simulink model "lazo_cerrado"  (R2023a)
settings: Solver=VariableStepAuto  StartTime=0.0  StopTime=10.0  RelTol=1e-3
libraries: visiontextngfix x6, slpidlib x3

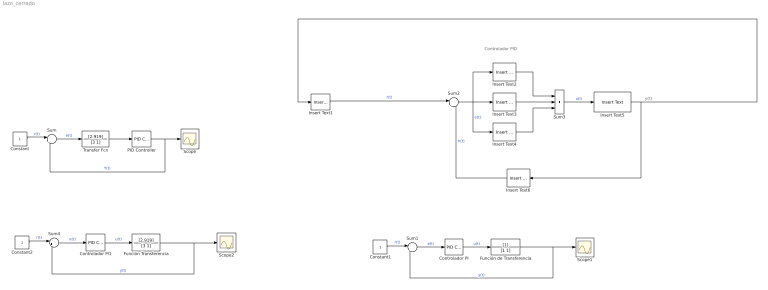
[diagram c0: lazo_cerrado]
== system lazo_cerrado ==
  note: Controlador PID
  note: y(t)
  Constant : Constant
  Constant1 : Constant
  Constant2 : Constant
  Controlador PI : slpidlib/PID Controller  Controller=PI  Form=Parallel  TimeDomain=Continuous-time  UseExternalTs=off  SampleTime=-1  IntegratorMethod=Forward Euler  FilterMethod=Forward Euler  ControllerParametersSource=internal  P=1  I=1  UseKiTs=off  D=0  N=100  UseFilter=on  TunerSelectOption=Transfer Function Based (PID Tuner App)  InitialConditionSource=internal  InitialConditionForIntegrator=0  InitialConditionForFilter=0  DifferentiatorICPrevScaledInput=0  ExternalReset=none  TrackingMode=off  Kt=1  LimitOutput=off  SatLimitsSource=internal  UpperSaturationLimit=inf  LowerSaturationLimit=-inf  LinearizeAsGain=on  AntiWindupMode=none  Kb=1  LimitIntegrator=off  UpperIntegratorSaturationLimit=inf  LowerIntegratorSaturationLimit=-inf  POutMin=[]  POutMax=[]  IOutMin=[]  IOutMax=[]  DOutMin=[]  DOutMax=[]  NOutMin=[]  NOutMax=[]  SumOutMin=[]  SumOutMax=[]  SaturationOutMin=[]  SaturationOutMax=[]  PParamMin=[]  PParamMax=[]  IParamMin=[]  IParamMax=[]  DParamMin=[]  DParamMax=[]  NParamMin=[]  NParamMax=[]  KbParamMin=[]  KbParamMax=[]  KtParamMin=[]  KtParamMax=[]  KbOutMin=[]  KbOutMax=[]  KtOutMin=[]  KtOutMax=[]  IntegratorOutMin=[]  IntegratorOutMax=[]  FilterOutMin=[]  FilterOutMax=[]  SumI1OutMin=[]  SumI1OutMax=[]  SumI2OutMin=[]  SumI2OutMax=[]  SumI3OutMin=[]  SumI3OutMax=[]  SumI4OutMin=[]  SumI4OutMax=[]  SumDOutMin=[]  SumDOutMax=[]  DifferentiatorOutMin=[]  DifferentiatorOutMax=[]  FilterDiffOutCoefMin=[]  FilterDiffOutCoefMax=[]  ReciprocalOutMin=[]  ReciprocalOutMax=[]  SumDenOutMin=[]  SumDenOutMax=[]  SumNumOutMin=[]  SumNumOutMax=[]  DivideOutMin=[]  DivideOutMax=[]  UdiffTsProdOutMin=[]  UdiffTsProdOutMax=[]  NTsProdOutMin=[]  NTsProdOutMax=[]  UintegralTsProdOutMin=[]  UintegralTsProdOutMax=[]  UngainTsProdOutMin=[]  UngainTsProdOutMax=[]  ClampingZeroOutDataTypeStr=Inherit: Inherit via back propagation  ClampingZeroOutMin=[]  ClampingZeroOutMax=[]  FilterDenConstantOutDataTypeStr=Inherit: Inherit via back propagation  FilterDenConstantOutMin=[]  FilterDenConstantOutMax=[]  PCopyOutDataTypeStr=Inherit: Inherit via back propagation  PCopyOutMin=[]  PCopyOutMax=[]  NCopyOutDataTypeStr=Inherit: Inherit via back propagation  NCopyOutMin=[]  NCopyOutMax=[]  IntegratorContinuousStateAttributes=''  IntegratorStateMustResolveToSignalObject=off  IntegratorRTWStateStorageClass=Auto  FilterContinuousStateAttributes=''  FilterStateMustResolveToSignalObject=off  FilterRTWStateStorageClass=Auto  ParallelPVariant=InternalParameters  IdealPVariant=Disabled  IVariant=InternalParameters  DVariant=Disabled  IntegratorVariant=Continuous  SatVariant=Disabled  AWVariant=Passthrough  PCopyVariant=Disabled  TRVariant=Disabled  FdbkBlocksVariant=Forward  IdealPFdbkVariant=Disabled  SatFdbkVariant=Disabled  DerivativeFilterVariant=Disabled  NVariant=Disabled  NCopyVariant=Disabled_SignalSpec  FilterICVariant=Disabled  IntegratorICVariant=InternalICs  ExternalResetVariant=Disabled  TRSumVariant=Passthrough  SumFdbkVariant=Disabled  SumVariant=Sum_PI  TsampFilterVariant=InternalTs  TsampNgainVariant=Passthrough  TsampIntegralVariant=Disabled_SignalSpec  ExternalSaturationOutDataTypeStr=Inherit: Same as second input
  Controlador PI1 : slpidlib/PID Controller  Controller=PI  Form=Parallel  TimeDomain=Continuous-time  UseExternalTs=off  SampleTime=-1  IntegratorMethod=Forward Euler  FilterMethod=Forward Euler  ControllerParametersSource=internal  P=1  I=1  UseKiTs=off  D=0  N=100  UseFilter=on  TunerSelectOption=Transfer Function Based (PID Tuner App)  InitialConditionSource=internal  InitialConditionForIntegrator=0  InitialConditionForFilter=0  DifferentiatorICPrevScaledInput=0  ExternalReset=none  TrackingMode=off  Kt=1  LimitOutput=off  SatLimitsSource=internal  UpperSaturationLimit=inf  LowerSaturationLimit=-inf  LinearizeAsGain=on  AntiWindupMode=none  Kb=1  LimitIntegrator=off  UpperIntegratorSaturationLimit=inf  LowerIntegratorSaturationLimit=-inf  POutMin=[]  POutMax=[]  IOutMin=[]  IOutMax=[]  DOutMin=[]  DOutMax=[]  NOutMin=[]  NOutMax=[]  SumOutMin=[]  SumOutMax=[]  SaturationOutMin=[]  SaturationOutMax=[]  PParamMin=[]  PParamMax=[]  IParamMin=[]  IParamMax=[]  DParamMin=[]  DParamMax=[]  NParamMin=[]  NParamMax=[]  KbParamMin=[]  KbParamMax=[]  KtParamMin=[]  KtParamMax=[]  KbOutMin=[]  KbOutMax=[]  KtOutMin=[]  KtOutMax=[]  IntegratorOutMin=[]  IntegratorOutMax=[]  FilterOutMin=[]  FilterOutMax=[]  SumI1OutMin=[]  SumI1OutMax=[]  SumI2OutMin=[]  SumI2OutMax=[]  SumI3OutMin=[]  SumI3OutMax=[]  SumI4OutMin=[]  SumI4OutMax=[]  SumDOutMin=[]  SumDOutMax=[]  DifferentiatorOutMin=[]  DifferentiatorOutMax=[]  FilterDiffOutCoefMin=[]  FilterDiffOutCoefMax=[]  ReciprocalOutMin=[]  ReciprocalOutMax=[]  SumDenOutMin=[]  SumDenOutMax=[]  SumNumOutMin=[]  SumNumOutMax=[]  DivideOutMin=[]  DivideOutMax=[]  UdiffTsProdOutMin=[]  UdiffTsProdOutMax=[]  NTsProdOutMin=[]  NTsProdOutMax=[]  UintegralTsProdOutMin=[]  UintegralTsProdOutMax=[]  UngainTsProdOutMin=[]  UngainTsProdOutMax=[]  ClampingZeroOutDataTypeStr=Inherit: Inherit via back propagation  ClampingZeroOutMin=[]  ClampingZeroOutMax=[]  FilterDenConstantOutDataTypeStr=Inherit: Inherit via back propagation  FilterDenConstantOutMin=[]  FilterDenConstantOutMax=[]  PCopyOutDataTypeStr=Inherit: Inherit via back propagation  PCopyOutMin=[]  PCopyOutMax=[]  NCopyOutDataTypeStr=Inherit: Inherit via back propagation  NCopyOutMin=[]  NCopyOutMax=[]  IntegratorContinuousStateAttributes=''  IntegratorStateMustResolveToSignalObject=off  IntegratorRTWStateStorageClass=Auto  FilterContinuousStateAttributes=''  FilterStateMustResolveToSignalObject=off  FilterRTWStateStorageClass=Auto  ParallelPVariant=InternalParameters  IdealPVariant=Disabled  IVariant=InternalParameters  DVariant=Disabled  IntegratorVariant=Continuous  SatVariant=Disabled  AWVariant=Passthrough  PCopyVariant=Disabled  TRVariant=Disabled  FdbkBlocksVariant=Forward  IdealPFdbkVariant=Disabled  SatFdbkVariant=Disabled  DerivativeFilterVariant=Disabled  NVariant=Disabled  NCopyVariant=Disabled_SignalSpec  FilterICVariant=Disabled  IntegratorICVariant=InternalICs  ExternalResetVariant=Disabled  TRSumVariant=Passthrough  SumFdbkVariant=Disabled  SumVariant=Sum_PI  TsampFilterVariant=InternalTs  TsampNgainVariant=Passthrough  TsampIntegralVariant=Disabled_SignalSpec  ExternalSaturationOutDataTypeStr=Inherit: Same as second input
  Función Transferencia : TransferFcn  Numerator=[2.919]  Denominator=[3 1]
  Función de Transferencia : TransferFcn  Denominator=[1 1]
  Insert Text1 : visiontextngfix/Insert Text  inputType=Obsolete  theText='K'  getTextLocFrom=Specify via dialog  textLoc=[1 1]  getTextColorFrom=Specify via dialog  textColor=[0 0 0]  getTextIntensityFrom=Specify via dialog  textIntensity=0  getTextOpacityFrom=Specify via dialog  textOpacity=1.0  dummyVar2=0  dummyVar3=0  dummyVar4=0  imagePorts=One multidimensional signal  isInputTransposed=off  fontFace=LucidaSansRegular  dummyVar1=0  blockFontSize=12  antiAliased=on
  Insert Text2 : visiontextngfix/Insert Text  inputType=Obsolete  theText='Kp'  getTextLocFrom=Specify via dialog  textLoc=[1 1]  getTextColorFrom=Specify via dialog  textColor=[0 0 0]  getTextIntensityFrom=Specify via dialog  textIntensity=0  getTextOpacityFrom=Specify via dialog  textOpacity=1.0  dummyVar2=0  dummyVar3=0  dummyVar4=0  imagePorts=One multidimensional signal  isInputTransposed=off  fontFace=LucidaSansRegular  dummyVar1=0  blockFontSize=12  antiAliased=on
  Insert Text3 : visiontextngfix/Insert Text  inputType=Obsolete  theText='Ki'  getTextLocFrom=Specify via dialog  textLoc=[1 1]  getTextColorFrom=Specify via dialog  textColor=[0 0 0]  getTextIntensityFrom=Specify via dialog  textIntensity=0  getTextOpacityFrom=Specify via dialog  textOpacity=1.0  dummyVar2=0  dummyVar3=0  dummyVar4=0  imagePorts=One multidimensional signal  isInputTransposed=off  fontFace=LucidaSansRegular  dummyVar1=0  blockFontSize=12  antiAliased=on
  Insert Text4 : visiontextngfix/Insert Text  inputType=Obsolete  theText='Kd'  getTextLocFrom=Specify via dialog  textLoc=[1 1]  getTextColorFrom=Specify via dialog  textColor=[0 0 0]  getTextIntensityFrom=Specify via dialog  textIntensity=0  getTextOpacityFrom=Specify via dialog  textOpacity=1.0  dummyVar2=0  dummyVar3=0  dummyVar4=0  imagePorts=One multidimensional signal  isInputTransposed=off  fontFace=LucidaSansRegular  dummyVar1=0  blockFontSize=12  antiAliased=on
  Insert Text5 : visiontextngfix/Insert Text  inputType=Obsolete  theText='Sistema'  getTextLocFrom=Specify via dialog  textLoc=[1 1]  getTextColorFrom=Specify via dialog  textColor=[0 0 0]  getTextIntensityFrom=Specify via dialog  textIntensity=0  getTextOpacityFrom=Specify via dialog  textOpacity=1.0  dummyVar2=0  dummyVar3=0  dummyVar4=0  imagePorts=One multidimensional signal  isInputTransposed=off  fontFace=LucidaSansRegular  dummyVar1=0  blockFontSize=12  antiAliased=on
  Insert Text6 : visiontextngfix/Insert Text  inputType=Obsolete  theText='Sensor'  getTextLocFrom=Specify via dialog  textLoc=[1 1]  getTextColorFrom=Specify via dialog  textColor=[0 0 0]  getTextIntensityFrom=Specify via dialog  textIntensity=0  getTextOpacityFrom=Specify via dialog  textOpacity=1.0  dummyVar2=0  dummyVar3=0  dummyVar4=0  imagePorts=One multidimensional signal  isInputTransposed=off  fontFace=LucidaSansRegular  dummyVar1=0  blockFontSize=12  antiAliased=on
  PID Controller : slpidlib/PID Controller  Controller=PI  Form=Parallel  TimeDomain=Continuous-time  UseExternalTs=off  SampleTime=-1  IntegratorMethod=Forward Euler  FilterMethod=Forward Euler  ControllerParametersSource=internal  P=1  I=1  UseKiTs=off  D=0  N=100  UseFilter=on  TunerSelectOption=Transfer Function Based (PID Tuner App)  InitialConditionSource=internal  InitialConditionForIntegrator=0  InitialConditionForFilter=0  DifferentiatorICPrevScaledInput=0  ExternalReset=none  TrackingMode=off  Kt=1  LimitOutput=off  SatLimitsSource=internal  UpperSaturationLimit=inf  LowerSaturationLimit=-inf  LinearizeAsGain=on  AntiWindupMode=none  Kb=1  LimitIntegrator=off  UpperIntegratorSaturationLimit=inf  LowerIntegratorSaturationLimit=-inf  POutMin=[]  POutMax=[]  IOutMin=[]  IOutMax=[]  DOutMin=[]  DOutMax=[]  NOutMin=[]  NOutMax=[]  SumOutMin=[]  SumOutMax=[]  SaturationOutMin=[]  SaturationOutMax=[]  PParamMin=[]  PParamMax=[]  IParamMin=[]  IParamMax=[]  DParamMin=[]  DParamMax=[]  NParamMin=[]  NParamMax=[]  KbParamMin=[]  KbParamMax=[]  KtParamMin=[]  KtParamMax=[]  KbOutMin=[]  KbOutMax=[]  KtOutMin=[]  KtOutMax=[]  IntegratorOutMin=[]  IntegratorOutMax=[]  FilterOutMin=[]  FilterOutMax=[]  SumI1OutMin=[]  SumI1OutMax=[]  SumI2OutMin=[]  SumI2OutMax=[]  SumI3OutMin=[]  SumI3OutMax=[]  SumI4OutMin=[]  SumI4OutMax=[]  SumDOutMin=[]  SumDOutMax=[]  DifferentiatorOutMin=[]  DifferentiatorOutMax=[]  FilterDiffOutCoefMin=[]  FilterDiffOutCoefMax=[]  ReciprocalOutMin=[]  ReciprocalOutMax=[]  SumDenOutMin=[]  SumDenOutMax=[]  SumNumOutMin=[]  SumNumOutMax=[]  DivideOutMin=[]  DivideOutMax=[]  UdiffTsProdOutMin=[]  UdiffTsProdOutMax=[]  NTsProdOutMin=[]  NTsProdOutMax=[]  UintegralTsProdOutMin=[]  UintegralTsProdOutMax=[]  UngainTsProdOutMin=[]  UngainTsProdOutMax=[]  ClampingZeroOutDataTypeStr=Inherit: Inherit via back propagation  ClampingZeroOutMin=[]  ClampingZeroOutMax=[]  FilterDenConstantOutDataTypeStr=Inherit: Inherit via back propagation  FilterDenConstantOutMin=[]  FilterDenConstantOutMax=[]  PCopyOutDataTypeStr=Inherit: Inherit via back propagation  PCopyOutMin=[]  PCopyOutMax=[]  NCopyOutDataTypeStr=Inherit: Inherit via back propagation  NCopyOutMin=[]  NCopyOutMax=[]  IntegratorContinuousStateAttributes=''  IntegratorStateMustResolveToSignalObject=off  IntegratorRTWStateStorageClass=Auto  FilterContinuousStateAttributes=''  FilterStateMustResolveToSignalObject=off  FilterRTWStateStorageClass=Auto  ParallelPVariant=InternalParameters  IdealPVariant=Disabled  IVariant=InternalParameters  DVariant=Disabled  IntegratorVariant=Continuous  SatVariant=Disabled  AWVariant=Passthrough  PCopyVariant=Disabled  TRVariant=Disabled  FdbkBlocksVariant=Forward  IdealPFdbkVariant=Disabled  SatFdbkVariant=Disabled  DerivativeFilterVariant=Disabled  NVariant=Disabled  NCopyVariant=Disabled_SignalSpec  FilterICVariant=Disabled  IntegratorICVariant=InternalICs  ExternalResetVariant=Disabled  TRSumVariant=Passthrough  SumFdbkVariant=Disabled  SumVariant=Sum_PI  TsampFilterVariant=InternalTs  TsampNgainVariant=Passthrough  TsampIntegralVariant=Disabled_SignalSpec  ExternalSaturationOutDataTypeStr=Inherit: Same as second input
  Scope : Scope
  Scope1 : Scope
  Scope2 : Scope
  Sum{,1..2,4} (4 alike) : Sum  Inputs=|+-
  Sum3 : Sum  Inputs=+++
  Transfer Fcn : TransferFcn  Numerator=[2.919]  Denominator=[3 1]
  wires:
  Sum/1 -> Transfer Fcn/1  "e(t)"
  Constant/1 -> Sum/1  "r(t)"
  Transfer Fcn/1 -> PID Controller/1
  PID Controller/1 -> Sum/2, Scope/1  "Y(t)"
  Constant1/1 -> Sum1/1  "r(t)"
  Sum1/1 -> Controlador PI/1  "e(t)"
  Controlador PI/1 -> Función de Transferencia/1  "u(t)"
  Insert Text1/1 -> Sum2/1  "r(t)"
  Sum2/1 -> Insert Text4/1, Insert Text2/1, Insert Text3/1  "e(t)"
  Insert Text2/1 -> Sum3/1
  Insert Text3/1 -> Sum3/2
  Insert Text4/1 -> Sum3/3
  Sum3/1 -> Insert Text5/1  "u(t)"
  Insert Text5/1 -> Insert Text1/1, Insert Text6/1
  Insert Text6/1 -> Sum2/2  "h(t)"
  Función de Transferencia/1 -> Sum1/2, Scope1/1  "y(t)"
  Sum4/1 -> Controlador PI1/1  "e(t)"
  Constant2/1 -> Sum4/1  "r(t)"
  Controlador PI1/1 -> Función Transferencia/1  "u(t)"
  Función Transferencia/1 -> Sum4/2, Scope2/1  "y(t)"
